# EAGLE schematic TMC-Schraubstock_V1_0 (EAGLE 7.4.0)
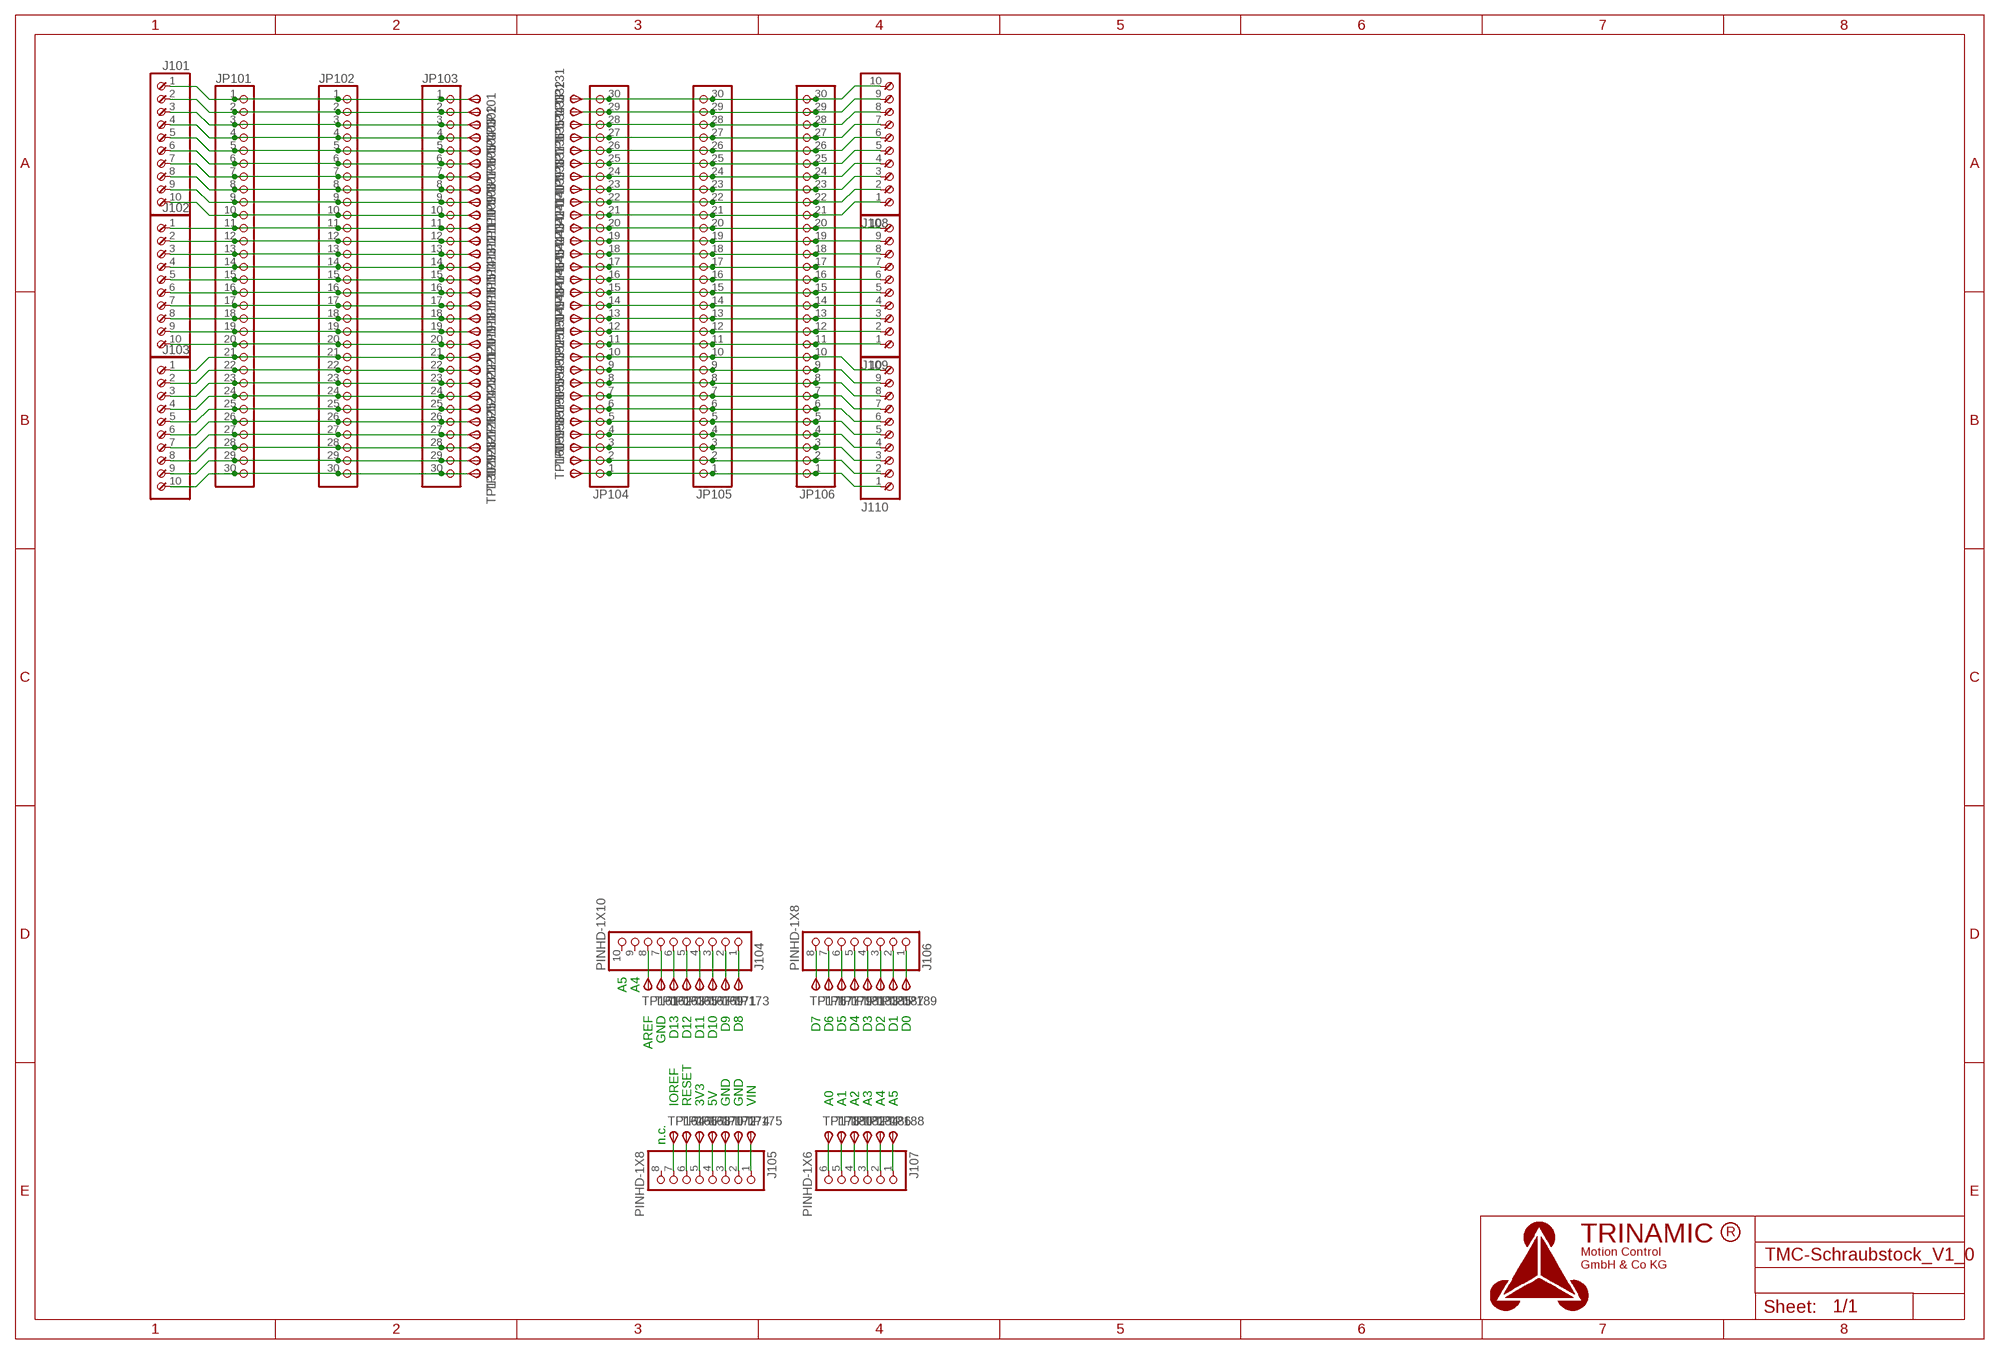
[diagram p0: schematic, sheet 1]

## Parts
J101  OSTVN10A150  [OSTVN10A150]
J102  OSTVN10A150  [OSTVN10A150]
J103  OSTVN10A150  [OSTVN10A150]
J104  PINHD-1X10  [1X10]
J105  PINHD-1X8  [1X08]
J106  PINHD-1X8  [1X08]
J107  PINHD-1X6  [1X06]
J108  OSTVN10A150  [OSTVN10A150]
J109  OSTVN10A150  [OSTVN10A150]
J110  OSTVN10A150  [OSTVN10A150]
JP101  PINHD-1X30  [1X30]
JP102  PINHD-1X30  [1X30]
JP103  PINHD-1X30  [1X30]
JP104  PINHD-1X30  [1X30]
JP105  PINHD-1X30  [1X30]
JP106  PINHD-1X30  [1X30]
TP101  TPSPAD1-13Y  [P1-13Y]
TP102  TPSPAD1-13Y  [P1-13Y]
TP103  TPSPAD1-13Y  [P1-13Y]
TP104  TPSPAD1-13Y  [P1-13Y]
TP105  TPSPAD1-13Y  [P1-13Y]
TP106  TPSPAD1-13Y  [P1-13Y]
TP107  TPSPAD1-13Y  [P1-13Y]
TP108  TPSPAD1-13Y  [P1-13Y]
TP109  TPSPAD1-13Y  [P1-13Y]
TP110  TPSPAD1-13Y  [P1-13Y]
TP111  TPSPAD1-13Y  [P1-13Y]
TP112  TPSPAD1-13Y  [P1-13Y]
TP113  TPSPAD1-13Y  [P1-13Y]
TP114  TPSPAD1-13Y  [P1-13Y]
TP115  TPSPAD1-13Y  [P1-13Y]
TP116  TPSPAD1-13Y  [P1-13Y]
TP117  TPSPAD1-13Y  [P1-13Y]
TP118  TPSPAD1-13Y  [P1-13Y]
TP119  TPSPAD1-13Y  [P1-13Y]
TP120  TPSPAD1-13Y  [P1-13Y]
TP121  TPSPAD1-13Y  [P1-13Y]
TP122  TPSPAD1-13Y  [P1-13Y]
TP123  TPSPAD1-13Y  [P1-13Y]
TP124  TPSPAD1-13Y  [P1-13Y]
TP125  TPSPAD1-13Y  [P1-13Y]
TP126  TPSPAD1-13Y  [P1-13Y]
TP127  TPSPAD1-13Y  [P1-13Y]
TP128  TPSPAD1-13Y  [P1-13Y]
TP129  TPSPAD1-13Y  [P1-13Y]
TP130  TPSPAD1-13Y  [P1-13Y]
TP131  TPSPAD1-13Y  [P1-13Y]
TP132  TPSPAD1-13Y  [P1-13Y]
TP133  TPSPAD1-13Y  [P1-13Y]
TP134  TPSPAD1-13Y  [P1-13Y]
TP135  TPSPAD1-13Y  [P1-13Y]
TP136  TPSPAD1-13Y  [P1-13Y]
TP137  TPSPAD1-13Y  [P1-13Y]
TP138  TPSPAD1-13Y  [P1-13Y]
TP139  TPSPAD1-13Y  [P1-13Y]
TP140  TPSPAD1-13Y  [P1-13Y]
TP141  TPSPAD1-13Y  [P1-13Y]
TP142  TPSPAD1-13Y  [P1-13Y]
TP143  TPSPAD1-13Y  [P1-13Y]
TP144  TPSPAD1-13Y  [P1-13Y]
TP145  TPSPAD1-13Y  [P1-13Y]
TP146  TPSPAD1-13Y  [P1-13Y]
TP147  TPSPAD1-13Y  [P1-13Y]
TP148  TPSPAD1-13Y  [P1-13Y]
TP149  TPSPAD1-13Y  [P1-13Y]
TP150  TPSPAD1-13Y  [P1-13Y]
TP151  TPSPAD1-13Y  [P1-13Y]
TP152  TPSPAD1-13Y  [P1-13Y]
TP153  TPSPAD1-13Y  [P1-13Y]
TP154  TPSPAD1-13Y  [P1-13Y]
TP155  TPSPAD1-13Y  [P1-13Y]
TP156  TPSPAD1-13Y  [P1-13Y]
TP157  TPSPAD1-13Y  [P1-13Y]
TP158  TPSPAD1-13Y  [P1-13Y]
TP159  TPSPAD1-13Y  [P1-13Y]
TP160  TPSPAD1-13Y  [P1-13Y]
TP161  TPSPAD1-13Y  [P1-13Y]
TP162  TPSPAD1-13Y  [P1-13Y]
TP163  TPSPAD1-13Y  [P1-13Y]
TP164  TPSPAD1-13Y  [P1-13Y]
TP165  TPSPAD1-13Y  [P1-13Y]
TP166  TPSPAD1-13Y  [P1-13Y]
TP167  TPSPAD1-13Y  [P1-13Y]
TP168  TPSPAD1-13Y  [P1-13Y]
TP169  TPSPAD1-13Y  [P1-13Y]
TP170  TPSPAD1-13Y  [P1-13Y]
TP171  TPSPAD1-13Y  [P1-13Y]
TP172  TPSPAD1-13Y  [P1-13Y]
TP173  TPSPAD1-13Y  [P1-13Y]
TP174  TPSPAD1-13Y  [P1-13Y]
TP175  TPSPAD1-13Y  [P1-13Y]
TP176  TPSPAD1-13Y  [P1-13Y]
TP177  TPSPAD1-13Y  [P1-13Y]
TP178  TPSPAD1-13Y  [P1-13Y]
TP179  TPSPAD1-13Y  [P1-13Y]
TP180  TPSPAD1-13Y  [P1-13Y]
TP181  TPSPAD1-13Y  [P1-13Y]
TP182  TPSPAD1-13Y  [P1-13Y]
TP183  TPSPAD1-13Y  [P1-13Y]
TP184  TPSPAD1-13Y  [P1-13Y]
TP185  TPSPAD1-13Y  [P1-13Y]
TP186  TPSPAD1-13Y  [P1-13Y]
TP187  TPSPAD1-13Y  [P1-13Y]
TP188  TPSPAD1-13Y  [P1-13Y]
TP189  TPSPAD1-13Y  [P1-13Y]

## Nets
N$1: J101.1 JP101.1 JP102.1 JP103.1 TP101.TP(PP)
N$2: J101.2 JP101.2 JP102.2 JP103.2 TP102.TP(PP)
N$3: J101.3 JP101.3 JP102.3 JP103.3 TP103.TP(PP)
N$4: J101.4 JP101.4 JP102.4 JP103.4 TP104.TP(PP)
N$5: J101.5 JP101.5 JP102.5 JP103.5 TP105.TP(PP)
N$6: J101.6 JP101.6 JP102.6 JP103.6 TP106.TP(PP)
N$7: J101.7 JP101.7 JP102.7 JP103.7 TP107.TP(PP)
N$8: J101.8 JP101.8 JP102.8 JP103.8 TP108.TP(PP)
N$9: J101.9 JP101.9 JP102.9 JP103.9 TP109.TP(PP)
N$10: J101.10 JP101.10 JP102.10 JP103.10 TP110.TP(PP)
N$11: J102.1 JP101.11 JP102.11 JP103.11 TP111.TP(PP)
N$12: J102.2 JP101.12 JP102.12 JP103.12 TP112.TP(PP)
N$13: J102.3 JP101.13 JP102.13 JP103.13 TP113.TP(PP)
N$14: J102.4 JP101.14 JP102.14 JP103.14 TP114.TP(PP)
N$15: J102.5 JP101.15 JP102.15 JP103.15 TP115.TP(PP)
N$16: J102.6 JP101.16 JP102.16 JP103.16 TP116.TP(PP)
N$17: J102.7 JP101.17 JP102.17 JP103.17 TP117.TP(PP)
N$18: J102.8 JP101.18 JP102.18 JP103.18 TP118.TP(PP)
N$19: J102.9 JP101.19 JP102.19 JP103.19 TP119.TP(PP)
N$20: J102.10 JP101.20 JP102.20 JP103.20 TP120.TP(PP)
N$21: J103.1 JP101.21 JP102.21 JP103.21 TP121.TP(PP)
N$22: J103.2 JP101.22 JP102.22 JP103.22 TP122.TP(PP)
N$23: J103.3 JP101.23 JP102.23 JP103.23 TP123.TP(PP)
N$24: J103.4 JP101.24 JP102.24 JP103.24 TP124.TP(PP)
N$25: J103.5 JP101.25 JP102.25 JP103.25 TP125.TP(PP)
N$26: J103.6 JP101.26 JP102.26 JP103.26 TP126.TP(PP)
N$27: J103.7 JP101.27 JP102.27 JP103.27 TP127.TP(PP)
N$28: J103.8 JP101.28 JP102.28 JP103.28 TP128.TP(PP)
N$29: J103.9 JP101.29 JP102.29 JP103.29 TP129.TP(PP)
N$30: J103.10 JP101.30 JP102.30 JP103.30 TP130.TP(PP)
N$31: J110.1 JP104.1 JP105.1 JP106.1 TP160.TP(PP)
N$32: J110.2 JP104.2 JP105.2 JP106.2 TP159.TP(PP)
N$33: J110.3 JP104.3 JP105.3 JP106.3 TP158.TP(PP)
N$34: J110.4 JP104.4 JP105.4 JP106.4 TP157.TP(PP)
N$35: J110.5 JP104.5 JP105.5 JP106.5 TP156.TP(PP)
N$36: J110.6 JP104.6 JP105.6 JP106.6 TP155.TP(PP)
N$37: J110.7 JP104.7 JP105.7 JP106.7 TP154.TP(PP)
N$38: J110.8 JP104.8 JP105.8 JP106.8 TP153.TP(PP)
N$39: J110.9 JP104.9 JP105.9 JP106.9 TP152.TP(PP)
N$40: J110.10 JP104.10 JP105.10 JP106.10 TP151.TP(PP)
N$41: J109.1 JP104.11 JP105.11 JP106.11 TP150.TP(PP)
N$42: J109.2 JP104.12 JP105.12 JP106.12 TP149.TP(PP)
N$43: J109.3 JP104.13 JP105.13 JP106.13 TP148.TP(PP)
N$44: J109.4 JP104.14 JP105.14 JP106.14 TP147.TP(PP)
N$45: J109.5 JP104.15 JP105.15 JP106.15 TP146.TP(PP)
N$46: J109.6 JP104.16 JP105.16 JP106.16 TP145.TP(PP)
N$47: J109.7 JP104.17 JP105.17 JP106.17 TP144.TP(PP)
N$48: J109.8 JP104.18 JP105.18 JP106.18 TP143.TP(PP)
N$49: J109.9 JP104.19 JP105.19 JP106.19 TP142.TP(PP)
N$50: J109.10 JP104.20 JP105.20 JP106.20 TP141.TP(PP)
N$51: J108.1 JP104.21 JP105.21 JP106.21 TP140.TP(PP)
N$52: J108.2 JP104.22 JP105.22 JP106.22 TP139.TP(PP)
N$53: J108.3 JP104.23 JP105.23 JP106.23 TP138.TP(PP)
N$54: J108.4 JP104.24 JP105.24 JP106.24 TP137.TP(PP)
N$55: J108.5 JP104.25 JP105.25 JP106.25 TP136.TP(PP)
N$56: J108.6 JP104.26 JP105.26 JP106.26 TP135.TP(PP)
N$57: J108.7 JP104.27 JP105.27 JP106.27 TP134.TP(PP)
N$58: J108.8 JP104.28 JP105.28 JP106.28 TP133.TP(PP)
N$59: J108.9 JP104.29 JP105.29 JP106.29 TP132.TP(PP)
N$60: J108.10 JP104.30 JP105.30 JP106.30 TP131.TP(PP)
N$62: J107.1 TP188.TP(PP)
N$63: J107.2 TP186.TP(PP)
N$64: J107.3 TP184.TP(PP)
N$65: J107.4 TP182.TP(PP)
N$66: J107.5 TP180.TP(PP)
N$67: J107.6 TP178.TP(PP)
N$68: J105.1 TP175.TP(PP)
N$69: J105.2 TP174.TP(PP)
N$70: J105.3 TP172.TP(PP)
N$71: J105.4 TP170.TP(PP)
N$72: J105.5 TP168.TP(PP)
N$73: J105.6 TP166.TP(PP)
N$74: J105.7 TP164.TP(PP)
N$76: J106.8 TP176.TP(PP)
N$77: J106.7 TP177.TP(PP)
N$78: J106.6 TP179.TP(PP)
N$79: J106.5 TP181.TP(PP)
N$80: J106.4 TP183.TP(PP)
N$81: J106.3 TP185.TP(PP)
N$82: J106.2 TP187.TP(PP)
N$83: J106.1 TP189.TP(PP)
N$86: J104.8 TP161.TP(PP)
N$87: J104.7 TP162.TP(PP)
N$88: J104.6 TP163.TP(PP)
N$89: J104.5 TP165.TP(PP)
N$90: J104.4 TP167.TP(PP)
N$91: J104.3 TP169.TP(PP)
N$92: J104.2 TP171.TP(PP)
N$93: J104.1 TP173.TP(PP)
Unconnected: J104.9 J104.10 J105.8

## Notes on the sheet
- A5 | A4
- AREF | GND | D13 | D12 | D11 | D10 | D9 | D8 | D7 | D6 | D5 | D4 | D3 | D2 | D1 | D0
- IOREF | RESET | 3V3 | 5V | GND | GND | VIN | A0 | A1 | A2 | A3 | A4 | A5
- n.c.

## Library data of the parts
J101-J103 J108-J110 = TMC-Schraubstock:OSTVN10A150: On Shore OSTVN10A150
J104 = TMC-Schraubstock:PINHD-1X10: PIN HEADER
J105 J106 = TMC-Schraubstock:PINHD-1X8: PIN HEADER
J107 = TMC-Schraubstock:PINHD-1X6: PIN HEADER
JP101-JP106 = pinhead:PINHD-1X30: PIN HEADER
TP101-TP189 = TMC-Schraubstock:TPS: TEST PIN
